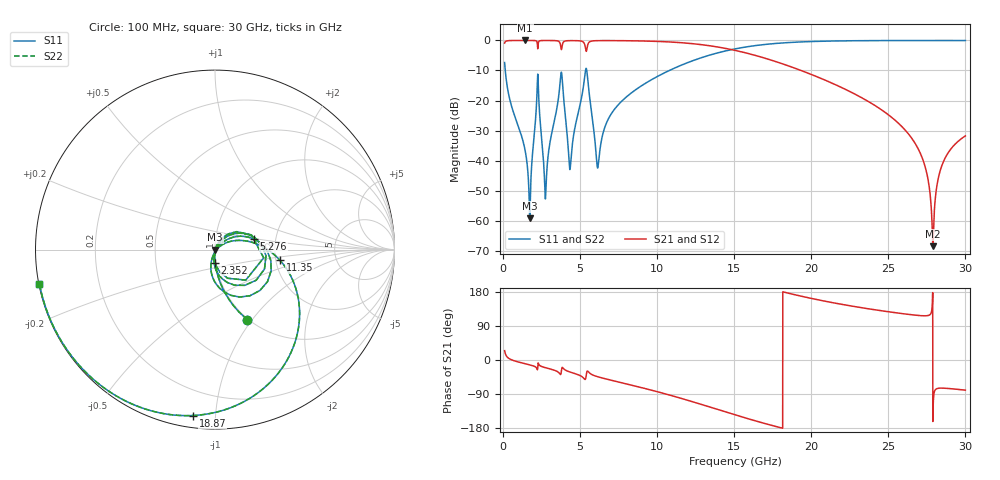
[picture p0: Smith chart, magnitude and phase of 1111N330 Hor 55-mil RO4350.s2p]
# GHz S MA R 50
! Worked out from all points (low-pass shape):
!   3201 points, 100 MHz to 30 GHz, reference 50 ohm
!   highest |S21| = -0.01 dB at 1.427 GHz (marker M1); lowest = -68.5 dB at 27.89 GHz (marker M2)
!   |S21| within 3 dB of the highest: start of sweep to 3.78 GHz; 5.434 GHz to 14.78 GHz (9.347 GHz wide, 92.5 % of centre)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
!   lowest |S11| = -59.3 dB at 1.726 GHz (marker M3), VSWR 1.00, Z = 50.1 - j0.0506 ohm
!   |S11| at or under -10 dB: 142.2 MHz to 5.351 GHz (5.208 GHz wide, 190 % of centre); 5.431 GHz to 10.79 GHz (5.357 GHz wide, 66.1 % of centre)
!   |S22| runs from -59.3 to 0.0 dB; largest |S21 - S12| = 0
!   S11 on the Smith chart (normalised r, x): 100 MHz: 0.99, -0.94; 2.352 GHz: 0.99, -0.14; 5.276 GHz: 1.55, +0.19; 11.35 GHz: 2.11, -0.29; 18.87 GHz: 0.06, -0.87; 30 GHz: 0.00, -0.10
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0.1  0.4288 -65.3  0.9032 24.6  0.9032 24.6  0.4288 -65.3
1.426813  0.01498 -96.9  0.999 -9.7  0.999 -9.7  0.01498 -96.9
1.725812  0.00109 -27.6  0.9987 -12.8  0.9987 -12.8  0.00109 -27.6
2.164969  0.08248 56.4  0.978 -20.6  0.978 -20.6  0.08248 56.4
2.351844  0.07257 -89.5  0.9798 -13.3  0.9798 -13.3  0.07257 -89.5
2.762969  0.002603 8.9  0.9974 -20.4  0.9974 -20.4  0.002603 8.9
3.734719  0.2478 11.2  0.8205 -38.2  0.8205 -38.2  0.2478 11.2
4.342062  0.007106 -21.9  0.9925 -31.7  0.9925 -31.7  0.007106 -21.9
5.089563  0.1106 36.1  0.9729 -43.1  0.9729 -43.1  0.1106 36.1
5.276438  0.2261 14.8  0.8819 -50.0  0.8819 -50.0  0.2261 14.8
6.15475  0.007741 -23.8  0.9921 -44.4  0.9921 -44.4  0.007741 -23.8
7.173219  0.06845 32.0  0.9933 -54.9  0.9933 -54.9  0.06845 32.0
10.06978  0.2559 4.9  0.9621 -84.3  0.9621 -84.3  0.2559 4.9
11.34988  0.3671 -9.4  0.925 -98.8  0.925 -98.8  0.3671 -9.4
15.05  0.7228 -55.0  0.6836 -144.6  0.6836 -144.6  0.7228 -55.0
18.87159  0.9324 -97.6  0.35 172.8  0.35 172.8  0.9324 -97.6
20.03956  0.9592 -108.2  0.2691 162.2  0.2691 162.2  0.9592 -108.2
25.01978  0.9953 -143.5  0.05748 127.2  0.05748 127.2  0.9953 -143.5
27.10344  0.9969 -155.0  0.01274 117.0  0.01274 117.0  0.9969 -155.0
27.88831  0.997 -159.0  0.000377 -162.3  0.000377 -162.3  0.997 -159.0
28.53303  0.9969 -162.2  0.009054 -74.2  0.009054 -74.2  0.9969 -162.2
30  0.9966 -169.1  0.0258 -79.6  0.0258 -79.6  0.9966 -169.1
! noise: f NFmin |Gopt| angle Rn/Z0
0.1  0.0006833  0.7415  1.976  0.0005298
3.417  0.02065  0.7153  24.9  0.01368
6.743  0.0229  0.5568  47.71  0.007867
10.06  0.02596  0.4749  64.97  0.00628
13.39  0.03731  0.5333  80.42  0.008778
16.7  0.05862  0.6481  96.96  0.0147
20.03  0.106  0.7845  115.7  0.02966
23.35  0.2445  0.9008  134.9  0.08053
26.67  1.259  0.9796  152.9  0.7857
30  1.023  0.9743  169  0.08612
